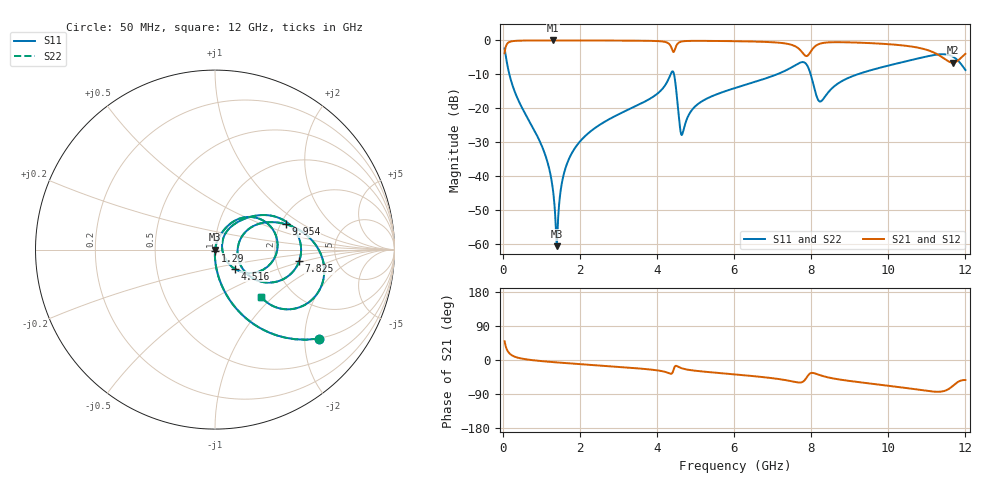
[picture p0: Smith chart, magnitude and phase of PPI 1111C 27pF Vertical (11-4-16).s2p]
# GHz S MA R 50
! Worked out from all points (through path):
!   1601 points, 50 MHz to 12 GHz, reference 50 ohm
!   highest |S21| = -0.01 dB at 1.312 GHz (marker M1); lowest = -6.6 dB at 11.67 GHz (marker M2)
!   group delay of S21, straight-line fit = 19.6 ps
!   lowest |S11| = -60.6 dB at 1.402 GHz (marker M3), VSWR 1.00, Z = 50.1 - j0.00925 ohm
!   |S11| at or under -10 dB: 173.5 MHz to 4.354 GHz (4.181 GHz wide, 185 % of centre); 4.444 GHz to 7.109 GHz (2.665 GHz wide, 46.1 % of centre); 7.987 GHz to 9.2 GHz (1.213 GHz wide, 14.1 % of centre)
!   |S22| runs from -60.6 to -2.4 dB; largest |S21 - S12| = 0
!   S11 on the Smith chart (normalised r, x): 50 MHz: 0.99, -2.34; 1.29 GHz: 1.00, -0.01; 4.516 GHz: 1.21, -0.26; 7.825 GHz: 2.71, -0.45; 9.954 GHz: 2.13, +0.73; 12 GHz: 1.39, -0.84
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0.05  0.761 -40.7  0.6486 49.3  0.6486 49.3  0.761 -40.7
0.2665938  0.2078 -79.1  0.9777 10.8  0.9777 10.8  0.2078 -79.1
1.043344  0.02548 -91.4  0.9988 -3.3  0.9988 -3.3  0.02548 -91.4
1.289813  0.007195 -88.3  0.999 -5.4  0.999 -5.4  0.007195 -88.3
1.312219  0.005734 -86.5  0.999 -5.6  0.999 -5.6  0.005734 -86.5
1.401844  0.0009316 -5.7  0.999 -6.3  0.999 -6.3  0.0009316 -5.7
1.618437  0.01258 77.4  0.9988 -8.0  0.9988 -8.0  0.01258 77.4
2.044156  0.03441 76.9  0.9981 -11.2  0.9981 -11.2  0.03441 76.9
4.038312  0.1691 59.3  0.9766 -27.8  0.9766 -27.8  0.1691 59.3
4.396813  0.3487 12.7  0.7293 -34.4  0.7293 -34.4  0.3487 12.7
4.516312  0.1522 -44.3  0.8632 -16.0  0.8632 -16.0  0.1522 -44.3
4.658219  0.04151 17.9  0.9676 -22.3  0.9676 -22.3  0.04151 17.9
5.046594  0.1136 57.3  0.9858 -28.9  0.9858 -28.9  0.1136 57.3
6.025  0.199 50.5  0.9746 -38.1  0.9746 -38.1  0.199 50.5
7.436594  0.385 28.3  0.8785 -54.9  0.8785 -54.9  0.385 28.3
7.824969  0.4733 -7.8  0.6117 -54.0  0.6117 -54.0  0.4733 -7.8
8.019156  0.273 -36.9  0.7268 -34.0  0.7268 -34.0  0.273 -36.9
8.243219  0.1261 0.4  0.9007 -40.5  0.9007 -40.5  0.1261 0.4
9.953563  0.4192 19.7  0.8851 -67.2  0.8851 -67.2  0.4192 19.7
10.01331  0.4275 18.9  0.8803 -68.0  0.8803 -68.0  0.4275 18.9
11.67137  0.578 -33.2  0.4704 -68.5  0.4704 -68.5  0.578 -33.2
12  0.3669 -45.6  0.6344 -52.9  0.6344 -52.9  0.3669 -45.6
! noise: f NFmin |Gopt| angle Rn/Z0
0.05  0.0003498  0.8591  1.009  0.0005314
1.372  0.003501  0.6544  6.201  0.001925
2.701  0.006112  0.6208  11.7  0.002978
4.031  0.01802  0.7903  17.72  0.01729
5.36  0.01626  0.7093  23.24  0.01058
6.682  0.02291  0.7426  28.63  0.01679
8.012  0.1651  0.953  34.79  0.7188
9.341  0.04047  0.799  39.57  0.03699
10.67  0.07412  0.8729  44.88  0.1075
12  0.2345  0.954  50.18  0.9419
